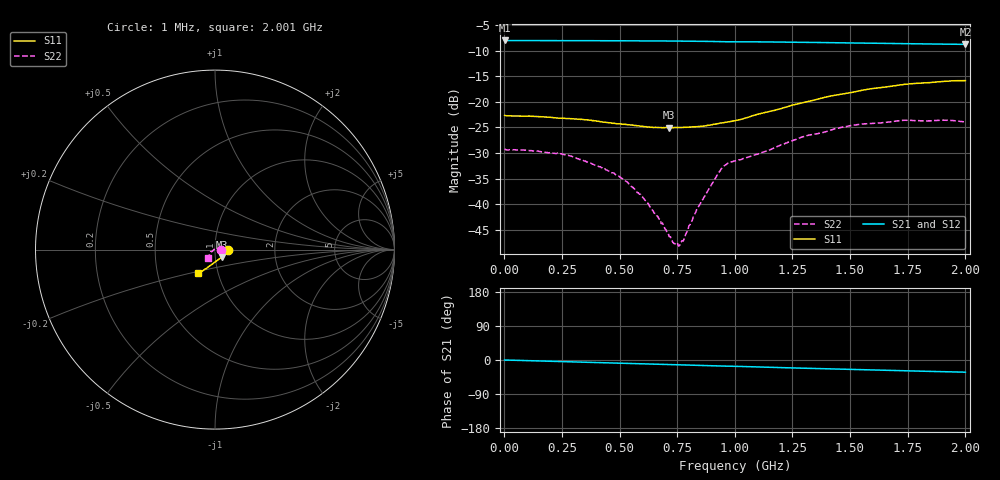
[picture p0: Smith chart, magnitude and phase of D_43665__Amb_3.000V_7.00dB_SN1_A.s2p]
! device id: 43665_
! dir: \\malibu\benchdata\1_engineers\tn_data\43665_75ohm\new\sparar\43665_\amb\3p000v\7p00db
! Serial: 1
! Insertion: A
! Temp: Amb
! VDD: 3.000V
! Attenuation Step: 7.00dB
! IDD: 1.455133e+00mA
! FILE NAME
! DATE 03-27-2009 08:35:05
! CORRECTED  DATA
#  Hz  S  RI  R  75
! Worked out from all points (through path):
!   401 points, 1 MHz to 2.001 GHz, reference 75 ohm
!   highest |S21| = -8.04 dB at 1 MHz (marker M1); lowest = -8.8 dB at 2.001 GHz (marker M2)
!   group delay of S21, straight-line fit = 45.4 ps
!   lowest |S11| = -25.1 dB at 716 MHz (marker M3), VSWR 1.12, Z = 80.4 - j6.76 ohm
!   |S11| at or under -10 dB: start of sweep to end of sweep
!   |S22| runs from -48.1 to -23.6 dB; largest |S21 - S12| = 0.0014
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1000000  0.0737 -0.000851  0.3963 -0.000699  0.3963 -0.00074  0.0347 -0.000177
2.41e8  0.0682 -0.0118  0.3942 -0.0271  0.3944 -0.0272  0.0301 0.00826
3.36e8  0.0654 -0.0168  0.3929 -0.038  0.3931 -0.038  0.0248 0.0109
4.66e8  0.0572 -0.0238  0.3904 -0.0527  0.3905 -0.0528  0.0173 0.0106
5.26e8  0.0533 -0.028  0.3887 -0.0596  0.3889 -0.0597  0.0137 0.00991
6.01e8  0.0471 -0.0332  0.3864 -0.0677  0.3865 -0.0679  0.00753 0.00896
6.71e8  0.0408 -0.0385  0.3844 -0.0757  0.3844 -0.0758  0.00349 0.00629
7.16e8  0.0368 -0.0419  0.3829 -0.0808  0.3829 -0.0808  0.00102 0.00472
7.36e8  0.0351 -0.0438  0.3822 -0.0832  0.3822 -0.0831  -0.000483 0.00413
7.51e8  0.0338 -0.0449  0.3815 -0.0848  0.3816 -0.0849  -0.00203 0.00367
7.66e8  0.0321 -0.046  0.3809 -0.0866  0.3809 -0.0866  -0.00312 0.00288
7.86e8  0.0303 -0.0477  0.3801 -0.089  0.3801 -0.089  -0.00487 0.00129
8.46e8  0.0236 -0.0524  0.3772 -0.0959  0.3771 -0.0958  -0.00916 -0.00352
9.31e8  0.0128 -0.0601  0.3714 -0.1049  0.3716 -0.1046  -0.0173 -0.0109
9.61e8  0.00997 -0.0623  0.3698 -0.1068  0.3699 -0.1066  -0.0219 -0.0107
1.001e9  0.00556 -0.0651  0.3687 -0.11  0.3689 -0.1099  -0.0243 -0.0105
1.336e9  -0.0366 -0.0961  0.3506 -0.1436  0.3512 -0.1436  -0.0339 -0.034
1.506e9  -0.0567 -0.1094  0.3394 -0.1583  0.3398 -0.1587  -0.0384 -0.0444
1.671e9  -0.0728 -0.1206  0.3286 -0.1712  0.3286 -0.1719  -0.0399 -0.0494
1.741e9  -0.0789 -0.1253  0.324 -0.1763  0.3241 -0.1772  -0.0405 -0.0523
1.911e9  -0.0894 -0.1306  0.313 -0.1875  0.3127 -0.1876  -0.0422 -0.0509
2.001e9  -0.0924 -0.1317  0.3074 -0.193  0.3063 -0.1939  -0.0408 -0.0486
